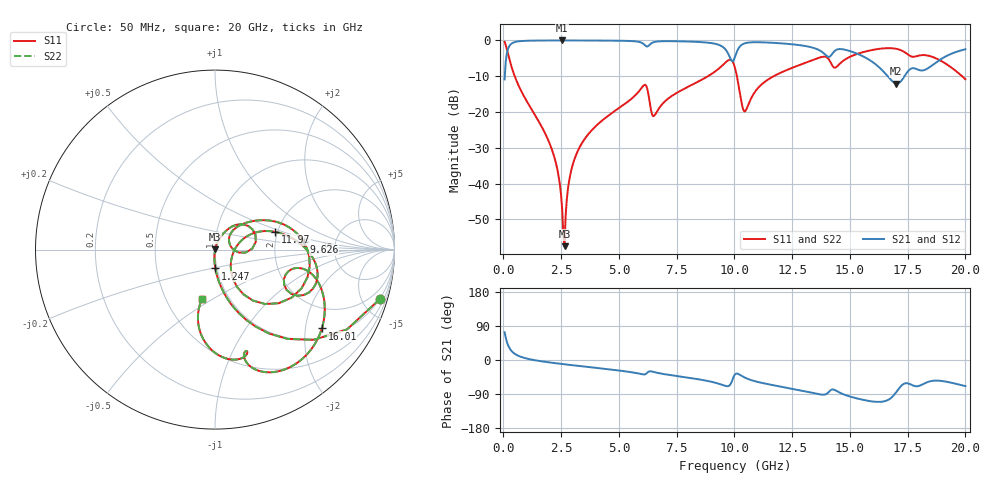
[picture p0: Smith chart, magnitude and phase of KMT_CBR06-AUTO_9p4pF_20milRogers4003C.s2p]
! Data measured by Modelithics Inc. support@modelithics.com 813-866-6335
! KEMET CBR06-AUTO 9.4pF, Pad Width= 0.851mm, Pad Length= 0.64mm, Pad Gap= 0.62mm, 20mil Rogers 4003C substrate Data, January 2022
# hz S ma R 50
! 2 Port Network Data from SP1.SP block
! freq  magS11  angS11  magS21  angS21  magS12  angS12  magS22  angS22
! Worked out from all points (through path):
!   401 points, 50 MHz to 20 GHz, reference 50 ohm
!   highest |S21| = -0.01 dB at 2.544 GHz (marker M1); lowest = -12.0 dB at 17.01 GHz (marker M2)
!   group delay of S21, straight-line fit = 13.5 ps
!   lowest |S11| = -57.5 dB at 2.643 GHz (marker M3), VSWR 1.00, Z = 50.1 + j0.0732 ohm
!   |S11| at or under -10 dB: 487.9 MHz to 8.852 GHz (8.364 GHz wide, 179 % of centre); 10.11 GHz to 11.7 GHz (1.593 GHz wide, 14.6 % of centre); 19.86 GHz to end of sweep
!   |S22| runs from -57.5 to -0.4 dB; largest |S21 - S12| = 0
!   S11 on the Smith chart (normalised r, x): 50 MHz: 0.98, -6.64; 1.247 GHz: 0.98, -0.21; 9.626 GHz: 2.92, +0.34; 11.97 GHz: 1.95, +0.44; 16.01 GHz: 1.27, -2.46; 20 GHz: 0.75, -0.45
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5e7  0.9584 -16.8  0.2851 73.2  0.2851 73.2  0.9584 -16.8
3.99125e8  0.3808 -69.2  0.9241 20.7  0.9241 20.7  0.3808 -69.2
1.247e9  0.105 -88.9  0.9937 0.7  0.9937 0.7  0.105 -88.9
2.194625e9  0.02395 -95.9  0.9988 -8.0  0.9988 -8.0  0.02395 -95.9
2.394125e9  0.01239 -95.3  0.9989 -9.5  0.9989 -9.5  0.01239 -95.3
2.54375e9  0.004353 -88.2  0.999 -10.6  0.999 -10.6  0.004353 -88.2
2.6435e9  0.00134 33.0  0.9989 -11.3  0.9989 -11.3  0.00134 33.0
2.94275e9  0.01574 72.8  0.9988 -13.5  0.9988 -13.5  0.01574 72.8
3.391625e9  0.03645 71.7  0.9981 -16.5  0.9981 -16.5  0.03645 71.7
6.084875e9  0.2373 28.3  0.8817 -38.3  0.8817 -38.3  0.2373 28.3
6.483875e9  0.08752 17.9  0.9402 -31.2  0.9402 -31.2  0.08752 17.9
6.73325e9  0.1125 43.3  0.9705 -34.8  0.9705 -34.8  0.1125 43.3
9.626e9  0.4957 5.0  0.7395 -68.6  0.7395 -68.6  0.4957 5.0
1.0025e10  0.4126 -47.3  0.5904 -37.9  0.5904 -37.9  0.4126 -47.3
1.047388e10  0.1032 -9.3  0.9161 -47.2  0.9161 -47.2  0.1032 -9.3
1.197012e10  0.3499 16.4  0.9133 -69.8  0.9133 -69.8  0.3499 16.4
1.336662e10  0.5286 -2.3  0.7964 -86.5  0.7964 -86.5  0.5286 -2.3
1.431425e10  0.418 -23.3  0.6994 -78.3  0.6994 -78.3  0.418 -23.3
1.601e10  0.7398 -36.4  0.492 -109.7  0.492 -109.7  0.7398 -36.4
1.670825e10  0.7797 -54.0  0.2977 -103.4  0.2977 -103.4  0.7797 -54.0
1.70075e10  0.7635 -62.8  0.2499 -84.9  0.2499 -84.9  0.7635 -62.8
2e10  0.2873 -104.8  0.7521 -69.0  0.7521 -69.0  0.2873 -104.8
